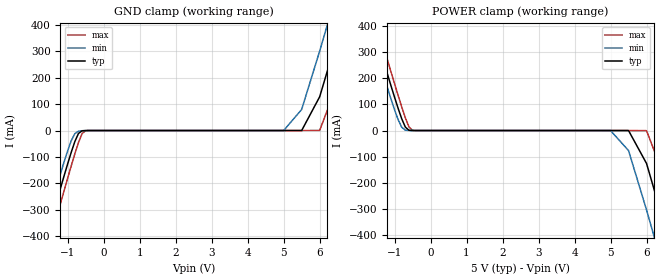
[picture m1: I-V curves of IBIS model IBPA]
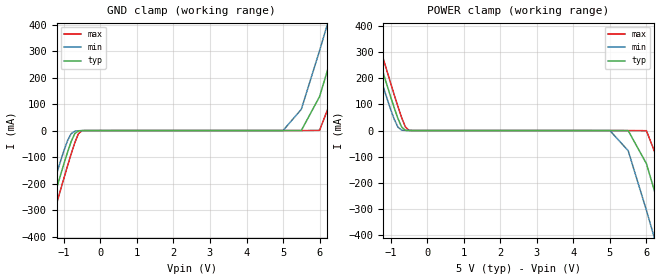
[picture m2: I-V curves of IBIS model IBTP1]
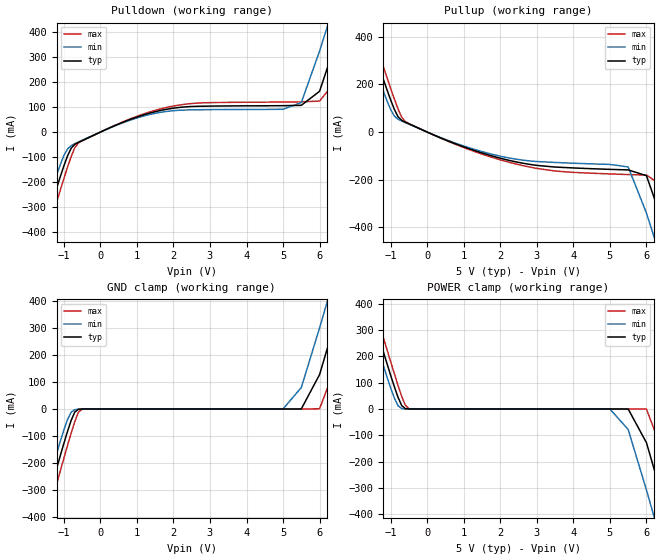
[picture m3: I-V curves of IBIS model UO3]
[IBIS Ver]   2.1
[File name]   apic21_0.ibs
[File Rev]   0.1
[Date]   4/14/99
[Source]   SEIKO EPSON CORP.
[Notes]
[Disclaimer]   Data is for modeling purposes only and is not guaranteed
   more disclaimer
[Copyright]   Copyright 1999 by SEIKO EPSON CORP.
[Component]   APIC21R00S
[Manufacturer] SEIKO EPSON CORP.
[Package]
|   QFP20-144
|   typ   min   max
R_pkg   111m   105m   117m
L_pkg   12.3nH   10.9nH  13.7nH
C_pkg   2.3pF   2.0pF   2.7pF
[Pin]   signal_name   model_name
1 VSS GND
2 PCI_AD23 UBPA
3 PCI_AD22 UBPA
4 PCI_AD21 UBPA
5 PCI_AD20 UBPA
6 PCI_AD19 UBPA
7 PCI_AD18 UBPA
8 PCI_AD17 UBPA
9 PCI_AD16 UBPA
10 VDD POWER
11 VSS GND
12 PCI_CBE2 IBPA
13 PCI_FRAME IBPA
14 PCI_IRDY IBPA
15 PCI_TRDY UOPA
16 PCI_DEVSEL UOPA
17 PCI_STOP UOPA
18 PCI_LOCK IBPA
19 PCI_PERR UOPA
20 PCI_SERR UOPA
21 PCI_PAR UBPA
22 PCI_CBE1 IBPA
23 VDD POWER
24 VSS GND
25 PCI_AD15 UBPA
26 PCI_AD14 UBPA
27 PCI_AD13 UBPA
28 PCI_AD12 UBPA
29 PCI_AD11 UBPA
30 PCI_AD10 UBPA
31 PCI_AD9 UBPA
32 PCI_AD8 UBPA
33 PCI_CBE0 IBPA
34 PCI_AD7 UBPA
35 PCI_AD6 UBPA
36 VDD POWER
37 VSS GND
38 PCI_AD5 UBPA
39 PCI_AD4 UBPA
40 PCI_AD3 UBPA
41 PCI_AD2 UBPA
42 PCI_AD1 UBPA
43 PCI_AD0 UBPA
44 VDD POWER
45 VSS GND
46 MASKN IBTP1
47 EEDO IBTP1
48 EEDI UO3
49 EESK UO3
50 EECS UO3
51 TOUTN UO3
52 TCLK UT3P1
53 VDD POWER
54 VSS GND
55 IRCN3 UO3
56 IRCN2 UO3
57 IRCN1 UO3
58 IRCN0 UO3
59 IRQ3 IBTP1
60 IRQ2 IBTP1
61 IRQ1 IBTP1
62 IRQ0 IBTP1
63 VDD POWER
64 VSS GND
65 TRESETN UO3
66 IORACKN UO3
67 IORREQN IBTP1
68 IORDY IBTP1
69 IOWN UO3
70 IORN UO3
71 BCLK UO3
72 VDD POWER
73 VSS GND
74 MWRN UO3
75 MRDN UO3
76 ROMCSN UO3
77 MEMCSN UO3
78 TD15 US4P1
79 TD14 US4P1
80 TD13 US4P1
81 TD12 US4P1
82 TD11 US4P1
83 TD10 US4P1
84 VDD POWER
85 VSS GND
86 TD9 US4P1
87 TD8 US4P1
88 TD7 US4P1
89 TD6 US4P1
90 TD5 US4P1
91 TD4 US4P1
92 TD3 US4P1
93 TD2 US4P1
94 TD1 US4P1
95 TD0 US4P1
96 VDD POWER
97 VSS GND
98 BHEN UO3
99 TA0 UO3
100 TA1 UO3
101 TA2 UO3
102 TA3 UO3
103 TA4 UO3
104 TA5 UO3
105 TA6 UO3
106 TA7 UO3
107 TA8 UO3
108 VDD POWER
109 VSS GND
110 TA_IOCSN0 UO3
111 TA_IOCSN1 UO3
112 TA_IOCSN2 UO3
113 TA_IOCSN3 UO3
114 TA_IOCSN4 UO3
115 TA_IOCSN5 UO3
116 TA_IOCSN6 UO3
117 TA_IOCSN7 UO3
118 VDD POWER
119 VSS GND
120 IOCSN7 UO3
121 IOCSN6 UO3
122 IOCSN5 UO3
123 IOCSN4 UO3
124 IOCSN3 UO3
125 IOCSN2 UO3
126 IOCSN1 UO3
127 IOCSN0 UO3
128 VDD POWER
129 VSS GND
130 PCI_INT UOPA
131 PCI_RST IBPA
132 PCI_CLK IBPA
133 VSS GND
134 PCI_AD31 UBPA
135 PCI_AD30 UBPA
136 PCI_AD29 UBPA
137 PCI_AD28 UBPA
138 PCI_AD27 UBPA
139 PCI_AD26 UBPA
140 PCI_AD25 UBPA
141 PCI_AD24 UBPA
142 PCI_CBE3 IBPA
143 PCI_IDSEL IBPA
144 VDD POWER
| Models and submodels in the file (7): IBPA (Input), IBTP1 (Input), UO3 (Output), UOPA (Output), UBPA (I/O), US4P1 (I/O), UT3P1 (I/O)
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[Model]   IBPA
Model_type   Input
Polarity   Non-Inverting
Vinh=2.0V
Vinl=0.8V
|   typ   min   max
C_comp   0   NA   NA
|   typ   min   max
[Voltage range]   5.0   4.5   5.5
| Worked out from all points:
|   GND clamp passes 1 mA (typ) near -0.58 V on its own axis
|   POWER clamp passes 1 mA (typ) near -0.60 V on its own axis
[GND_clamp]
|   Voltage   I(typ)   I(min)   I(max)
-10V      -4.607A    -4.528A    -4.688A
-1.7V     -460.6mA   -400.6mA   -521.8mA
-1.5V     -363.2mA   -304.7mA   -423.3mA
-900mV    -82.27mA   -38.72mA   -134mA
-700mV    -11.21mA   -2.502mA   -45.82mA
-500mV    -166.9uA   -220.4uA   -514.2uA
5V        307.6pA    28.74uA    220.4pA
5.5V      38.69uA    79.94mA    289.2pA
6V        128mA      301.2mA    669.1uA
6.5V      356.8mA    534.3mA    179.8mA
7V        592.7mA    770.6mA    413.7mA
10V       2.033A     2.206A     1.857A
[POWER_clamp]
|   Voltage   I(typ)   I(min)   I(max)
-10V      4.449A     4.374A     4.525A
-1.8V     498mA      440.5mA    556.5mA
-1.7V     450.8mA    393.8mA    508.8mA
-1.5V     356.8mA    301.2mA    413.8mA
-900mV    84.98mA    41.78mA    134.5mA
-500mV    38.69uA    28.74uA    670.2uA
5V        -482.9pA   -220.4uA   -397pA
5.5V      -166.9uA   -76.84mA   -467.2pA
6V        -126.4mA   -304.6mA   -514.1uA
6.5V      -363.1mA   -546.1mA   -180.9mA
7V        -607.7mA   -791.1mA   -423.2mA
10V       -2.101A    -2.28A     -1.92A
[Model]   IBTP1
Model_type   Input
Polarity   Non-Inverting
Vinh=2.0V
Vinl=0.8V
|   typ   min   max
C_comp   0   NA   NA
|   typ   min   max
[Voltage range]   5.0   4.5   5.5
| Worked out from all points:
|   GND clamp passes 1 mA (typ) near -0.57 V on its own axis
|   POWER clamp passes 1 mA (typ) near -0.60 V on its own axis
[GND_clamp]
|   Voltage   I(typ)   I(min)   I(max)
-10V      -4.608A    -4.528A    -4.688A
-1.7V     -460.7mA   -400.7mA   -521.9mA
-1.5V     -363.3mA   -304.8mA   -423.4mA
-900mV    -82.38mA   -38.82mA   -134.1mA
-700mV    -11.32mA   -2.606mA   -45.93mA
-500mV    -276.9uA   -320.4uA   -634uA
5V        307.6pA    38.74uA    -10uA
5.5V      48.69uA    79.96mA    289.2pA
6V        128mA      301.2mA    679.1uA
6.5V      356.8mA    534.3mA    179.9mA
7V        592.7mA    770.6mA    413.8mA
10V       2.033A     2.207A     1.857A
[POWER_clamp]
|   Voltage   I(typ)   I(min)   I(max)
-10V      4.449A     4.374A     4.525A
-1.8V     498mA      440.5mA    556.5mA
-1.7V     450.8mA    393.8mA    508.8mA
-1.5V     356.8mA    301.2mA    413.8mA
-900mV    84.99mA    41.8mA     134.5mA
-500mV    48.69uA    38.74uA    680.2uA
5V        -100uA     -320.4uA   -100uA
5.5V      -276.9uA   -76.94mA   -110uA
6V        -126.5mA   -304.7mA   -633.9uA
6.5V      -363.3mA   -546.2mA   -181mA
7V        -607.8mA   -791.2mA   -423.4mA
10V       -2.101A    -2.28A     -1.921A
[Model]   UO3
Model_type   Output
Polarity   Non-Inverting
|   typ   min   max
C_comp   0   NA   NA
|   typ   min   max
[Voltage range]   5.0   4.5   5.5
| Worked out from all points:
|   slope of the pulldown table from 0 to 0.75 V, typ, clamps not added: 16 ohm
|   slope of the pullup table from 0 to 0.75 V, typ, clamps not added: 15.7 ohm
|   GND clamp passes 1 mA (typ) near -0.58 V on its own axis
|   POWER clamp passes 1 mA (typ) near -0.60 V on its own axis
[Pulldown]
|   Voltage   I(typ)   I(min)   I(max)
-10V      -4.641A    -4.561A    -4.722A
-1.8V     -515.5mA   -455.3mA   -576.9mA
-1.5V     -368.9mA   -311.4mA   -428.4mA
-1V       -136.1mA   -94.55mA   -186.8mA
-700mV    -49.02mA   -46.59mA   -62.53mA
-500mV    -34.28mA   -33.03mA   -35.35mA
2V        95.77mA    85.67mA    104.3mA
5.5V      107.1mA    118.1mA    121.1mA
6V        163.3mA    324.3mA    124.1mA
6.5V      383.1mA    554.5mA    215.6mA
7V        616.7mA    789.1mA    443.8mA
10V       2.051A     2.22A      1.883A
[Pullup]
|   Voltage   I(typ)   I(min)   I(max)
-10V      4.425A     4.351A     4.5A
-1.9V     543.7mA    486.7mA    601.8mA
-1.6V     403.5mA    348.4mA    459.9mA
-1V       134.3mA    94.03mA    182.4mA
-700mV    49.17mA    46.54mA    62.68mA
-500mV    34.57mA    33.17mA    35.76mA
2.5V      -127.1mA   -115.2mA   -136.4mA
5.5V      -158.6mA   -146mA     -178.1mA
6V        -182.7mA   -339.6mA   -180.2mA
6.5V      -401.6mA   -579.4mA   -231.5mA
7V        -645.3mA   -824.9mA   -465mA
10V       -2.147A    -2.323A    -1.969A
[GND_clamp]
|   Voltage   I(typ)   I(min)   I(max)
-10V      -4.641A    -4.561A    -4.722A
-1.7V     -464.3mA   -404mA     -525.9mA
-1.5V     -366.3mA   -307.4mA   -426.7mA
-1.4V     -317.6mA   -259.6mA   -377.3mA
-900mV    -83.24mA   -39.38mA   -135.3mA
-500mV    -173.5uA   -229.2uA   -533.5uA
5V        319.4pA    28.04uA    231.5pA
5.5V      37.76uA    79.26mA    300.3pA
6V        127mA      299.3mA    653.9uA
6.5V      354.6mA    531.1mA    178.7mA
7V        589.2mA    766.1mA    411.3mA
10V       2.021A     2.194A     1.847A
[POWER_clamp]
|   Voltage   I(typ)   I(min)   I(max)
-10V      4.425A     4.35A      4.5A
-1.8V     495mA      437.8mA    553.2mA
-1.6V     401.3mA    345.2mA    458.5mA
-1.5V     354.6mA    299.3mA    411.3mA
-900mV    84.3mA     41.34mA    133.6mA
-500mV    37.76uA    28.04uA    654.9uA
5V        -471.3pA   -229.2uA   -385.8pA
5.5V      -173.5uA   -77.83mA   -456.1pA
6V        -127.7mA   -307.2mA   -533.4uA
6.5V      -366.2mA   -550.5mA   -182.5mA
7V        -612.5mA   -797.3mA   -426.6mA
10V       -2.116A    -2.297A    -1.935A
[Ramp]
|   V_typ   V_min   V_max
dV/dt_r   3.00/3.684e-10   2.70/3.571e-10   3.30/3.893e-10
dV/dt_f   3.00/3.854e-10   2.70/3.697e-10   3.30/3.850e-10
R_load = 5000ohm
